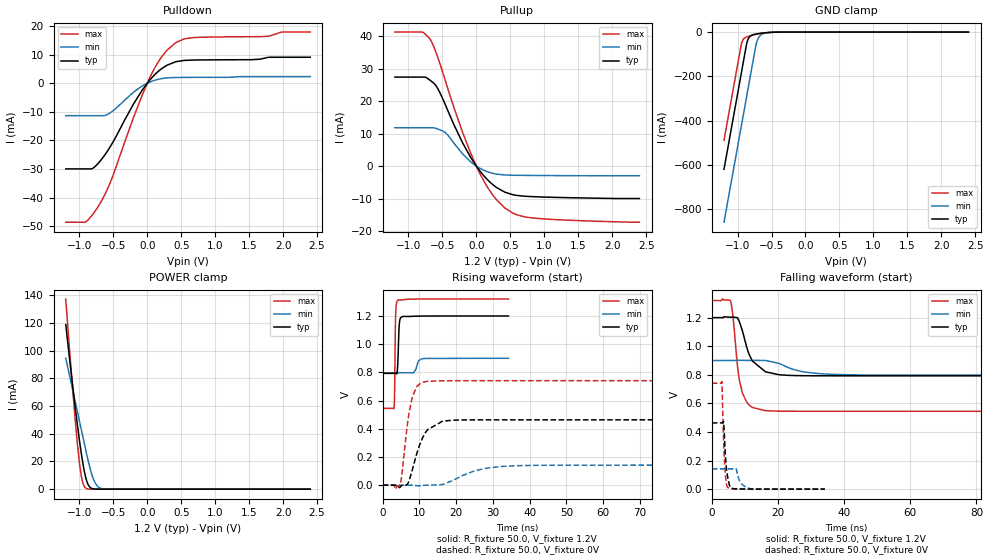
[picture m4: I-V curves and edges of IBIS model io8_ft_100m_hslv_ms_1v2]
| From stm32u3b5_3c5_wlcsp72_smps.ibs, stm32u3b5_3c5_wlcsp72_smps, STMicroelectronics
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[Model]   io8_ft_100m_hslv_ms_1v2
Model_type I/O
Polarity   Non-Inverting
Enable   Active-Low
| CAP_THRESHOLD on pad IOFT is "UDTCAPC" :
| Rising=30.0% of vddiom   Falling=70.0% of vddiom
| C_comp min and max val. don't necessarily correlate with the min and max pvt
| but are the smallest and greatest pad capacitance found.
| var   typ   min   max
C_comp   2.92730pF  2.86805pF  2.98035pF
|C_comp_pullup   1.66509pF  1.49588pF  1.80346pF
|C_comp_pulldown   1.26221pF  1.37217pF  1.17689pF
Vinl = 450.0mV
Vinh = 660.0mV
Vmeas = 600.0mV   | Reference voltage for timing measurements
Cref  = 50.0pF   | Timing specification test load capacitance value
Rref  = 1.0MOhm   | Timing specification test load resistance value
Vref  = 660.0mV   | Timing specification test load voltage
[Model Spec]
| TIME_THRESHOLD on pin ZIV11 is "CMOS" :
| Rising=50.0% of vdd   Falling=50.0% of vdd
Vinl 439.50000mV 331.50001mV 485.50000mV
Vinh 752.50000mV 552.50001mV 837.50000mV
| variable   typ   min   max
[Temperature Range] 25.0 130.0 -40.0
| variable   typ   min   max
[Voltage Range] 1.2V 900.0mV 1.32V
| variable   typ   min   max
[POWER Clamp Reference] 1.2V 900.0mV 1.32V
| variable   typ   min   max
[GND Clamp Reference] 0V 0V 0V
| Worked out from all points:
|   slope of the pulldown table from 0 to 0.18 V, typ, clamps not added: 40 ohm
|   slope of the pullup table from 0 to 0.18 V, typ, clamps not added: 40 ohm
|   GND clamp passes 1 mA (typ) near -0.50 V on its own axis
|   POWER clamp passes 1 mA (typ) near -0.83 V on its own axis
|   rising waveform, R_fixture 50.0, V_fixture 1.2V: 20-80 % time 332ps typ, 807ps min, 221ps max; typ from 0.793 V to 1.2 V
|   falling waveform, R_fixture 50.0, V_fixture 1.2V: 20-80 % time 4.34ns typ, 8.19ns min, 2.39ns max; typ from 1.2 V to 0.793 V
|   rising waveform, R_fixture 50.0, V_fixture 0V: 20-80 % time 3.69ns typ, 8.42ns min, 2.26ns max; typ from 0 V to 0.464 V
|   falling waveform, R_fixture 50.0, V_fixture 0V: 20-80 % time 930ps typ, 1.77ns min, 719ps max; typ from 0.464 V to 0 V
[POWER Clamp]
-1.2V     118.8mA    94.44mA    137.2mA
-1.09V    71.2mA     69.75mA    67.14mA
-1.02V    43.22mA    54.03mA    28.67mA
-990mV    32.26mA    47.3mA     15.78mA
-970mV    25.49mA    42.81mA    9.257mA
-940mV    16.45mA    36.08mA    3.257mA
-910mV    9.238mA    29.34mA    904.6uA
-860mV    2.387mA    18.53mA    87.46uA
-790mV    204.6uA    7.049mA    3.101uA
-730mV    21.91uA    2.041mA    176.4nA
-660mV    1.594uA    337.6uA    6.282nA
2.4V      0A         0A         0A
[GND Clamp]
-1.2V     -619mA     -857.5mA   -488.2mA
-950mV    -194mA     -432.5mA   -63.18mA
-930mV    -160mA     -398.5mA   -40.87mA
-870mV    -57.95mA   -296.5mA   -22.39mA
-840mV    -28.97mA   -245.5mA   -19.16mA
-800mV    -15.67mA   -177.5mA   -15.71mA
-730mV    -8.807mA   -59.89mA   -10.55mA
-700mV    -7.204mA   -30.66mA   -8.61mA
-660mV    -5.427mA   -13.83mA   -6.309mA
-580mV    -2.713mA   -4.125mA   -2.796mA
-380mV    -62.64uA   -240.2uA   -21.17uA
2.4V      834.9pA    121.9nA    346.5pA
| variable   typ   min   max
[Pullup Reference] 1.2V 900.0mV 1.32V
| variable   typ   min   max
[Pulldown Reference] 0V 0V 0V
[Pullup]
-1.2V     27.37mA    11.8mA     41.2mA
-800mV    27.37mA    11.8mA     41.2mA
-680mV    26.37mA    11.8mA     38.99mA
-580mV    24.24mA    11.5mA     34.13mA
-460mV    19.02mA    10.35mA    26.45mA
-200mV    7.047mA    3.687mA    10.21mA
0V        518.5fA    131.7pA    2.78fA
210mV     -5.089mA   -2.027mA   -7.926mA
420mV     -8mA       -2.709mA   -12.87mA
580mV     -8.947mA   -2.8mA     -14.83mA
790mV     -9.331mA   -2.845mA   -15.82mA
2.4V      -9.943mA   -2.948mA   -17.22mA
[Pulldown]
-1.2V     -29.93mA   -11.33mA   -48.55mA
-910mV    -29.93mA   -11.33mA   -48.48mA
-810mV    -29.8mA    -11.33mA   -46.03mA
-710mV    -27.65mA   -11.33mA   -42.6mA
-530mV    -21.58mA   -10.08mA   -33.79mA
-200mV    -7.157mA   -3.075mA   -11.82mA
40mV      1.18mA     424.7uA    2.081mA
220mV     5.228mA    1.661mA    9.479mA
420mV     7.512mA    2.016mA    14.19mA
670mV     8.097mA    2.046mA    15.93mA
1.78V     9.043mA    2.312mA    16.4mA
2.4V      9.076mA    2.312mA    17.87mA
[Ramp]
dV/dt_r 278.14129mV/3.68502ns 85.18546mV/8.15865ns 444.65552mV/2.22624ns
dV/dt_f 244.20998mV/3.83884ns 61.55655mV/8.16358ns 465.10808mV/2.31912ns
R_load = 50.0
| Removed startup time: 0s 0s 0s  .
| Removed end time: 34.25ns.
[Rising Waveform]
R_fixture   = 50.0
V_fixture   = 1.2V
V_fixture_min = 900.0mV
V_fixture_max = 1.32V
0s        793mV      797.4mV    544.8mV
3.1ns     793.1mV    797.4mV    547.9mV
3.25ns    793.2mV    797.4mV    652.9mV
3.45ns    793.4mV    797.4mV    1.105V
3.55ns    793.3mV    797.4mV    1.215V
4.1ns     850.5mV    797.4mV    1.311V
4.6ns     1.159V     797.4mV    1.314V
5.6ns     1.197V     797.4mV    1.316V
11.2ns    1.199V     897.9mV    1.32V
34.25ns   1.2V       899.9mV    1.32V
| Removed startup time: 0s 0s 0s  .
| Removed end time: 199.25ns.
[Falling Waveform]
R_fixture   = 50.0
V_fixture   = 1.2V
V_fixture_min = 900.0mV
V_fixture_max = 1.32V
0s        1.2V       900mV      1.32V
5.65ns    1.203V     900mV      1.318V
6.4ns     1.203V     900mV      1.21V
8.05ns    1.187V     902.2mV    809.6mV
9.3ns     1.105V     901mV      670.1mV
12.2ns    899.9mV    900.8mV    572.9mV
16.25ns   820.7mV    900.5mV    549.1mV
27.05ns   793.9mV    823.7mV    544.9mV
40.65ns   793mV      800.5mV    544.8mV
199.3ns   793mV      797.4mV    544.8mV
| Removed startup time: 0s 0s 0s  .
| Removed end time: 199.2ns.
[Rising Waveform]
R_fixture   = 50.0
V_fixture   = 0V
V_fixture_min = 0V
V_fixture_max = 0V
0s        4.608nV    136.5nV    3.237nV
4.75ns    -13.99mV   -1.446uV   7.223mV
6.85ns    11.59mV    -24.86uV   451.4mV
8ns       101.5mV    115.3uV    617.5mV
9.25ns    220.9mV    -3.472mV   697mV
12.2ns    393.2mV    -164.2uV   736.6mV
16.25ns   453.2mV    3.834mV    740.6mV
25.55ns   463.2mV    105mV      741mV
36.6ns    463.4mV    138.3mV    741mV
199.2ns   463.6mV    142mV      741.1mV
| Removed startup time: 0s 0s 0s  .
| Removed end time: 34.2ns.
[Falling Waveform]
R_fixture   = 50.0
V_fixture   = 0V
V_fixture_min = 0V
V_fixture_max = 0V
0s        463.6mV    142mV      741.1mV
3.05ns    463.9mV    142mV      753.4mV
3.6ns     468.1mV    142mV      320.8mV
3.85ns    357.9mV    142mV      195.1mV
4.35ns    167.2mV    142mV      49.81mV
4.9ns     72.29mV    142.1mV    10.71mV
7.25ns    2.303mV    147.1mV    1.278mV
8.4ns     1.782mV    58.81mV    659.7uV
11.2ns    583uV      5.937mV    178uV
34.2ns    298nV      54.43uV    87.07nV
